FUNCTION "CENTRATORE" : VOID
TITLE =COMANDO CENTRATORE
AUTHOR : D_T
FAMILY : DESTACK
NAME : CENTRAG
VERSION : 0.1

BEGIN
NETWORK
TITLE =Staz.di Centraggio: Comando sblocco
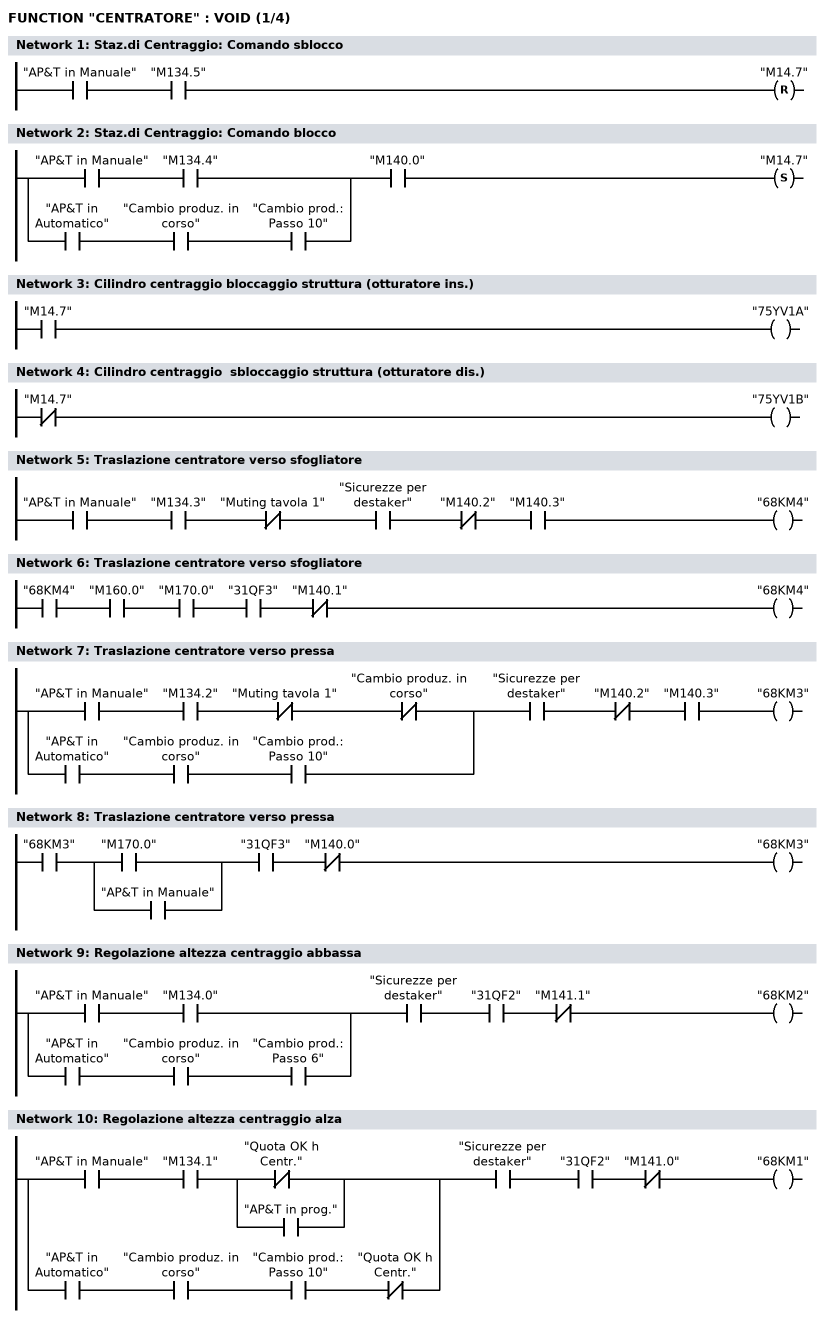
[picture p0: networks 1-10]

      U     "AP&T in Manuale";
      U     "M134.5";
      R     "M14.7";
NETWORK
TITLE =Staz.di Centraggio: Comando blocco

      U(    ;
      U     "AP&T in Manuale";
      U     "M134.4";
      O     ;
      U     "AP&T in Automatico";
      U     "Cambio produz. in corso";
      U     "Cambio prod.: Passo 10";
      )     ;
      U     "M140.0";
      S     "M14.7";
NETWORK
TITLE =Cilindro centraggio bloccaggio struttura (otturatore ins.)

      U     "M14.7";
//      U     "39SQ3"
      =     "75YV1A";
NETWORK
TITLE =Cilindro centraggio  sbloccaggio struttura (otturatore dis.)

      UN    "M14.7";
//      U     "39SQ1"
      =     "75YV1B";
NETWORK
TITLE =Traslazione centratore verso sfogliatore

      U     "AP&T in Manuale";
      U     "M134.3";
      UN    "Muting tavola 1";
      U     "Sicurezze per destaker";
      UN    "M140.2";
      U     "M140.3";
      =     "68KM4";
NETWORK
TITLE =Traslazione centratore verso sfogliatore

      U     "68KM4";
      U     "M160.0";
      U     "M170.0";
      U     "31QF3";
      UN    "M140.1";
      =     "68KM4";
NETWORK
TITLE =Traslazione centratore verso pressa

      U(    ;
      U     "AP&T in Manuale";
      U     "M134.2";
      UN    "Muting tavola 1";
      UN    "Cambio produz. in corso";
      O     ;
      U     "AP&T in Automatico";
      U     "Cambio produz. in corso";
      U     "Cambio prod.: Passo 10";
      )     ;
      U     "Sicurezze per destaker";
      UN    "M140.2";
      U     "M140.3";
      =     "68KM3";
NETWORK
TITLE =Traslazione centratore verso pressa

      U     "68KM3";
      U(    ;
      O     "M170.0";
      O     "AP&T in Manuale";
      )     ;
      U     "31QF3";
      UN    "M140.0";
      =     "68KM3";
NETWORK
TITLE =Regolazione altezza centraggio abbassa

      U(    ;
      U     "AP&T in Manuale";
      U     "M134.0";
      O     ;
      U     "AP&T in Automatico";
      U     "Cambio produz. in corso";
      U     "Cambio prod.: Passo 6";
      )     ;
      U     "Sicurezze per destaker";
      U     "31QF2";
      UN    "M141.1";
      =     "68KM2";
NETWORK
TITLE =Regolazione altezza centraggio alza

      U(    ;
      U     "AP&T in Manuale";
      U     "M134.1";
      U(    ;
      ON    "Quota OK h Centr.";
      O     "AP&T in prog.";
      )     ;
      O     ;
      U     "AP&T in Automatico";
      U     "Cambio produz. in corso";
      U     "Cambio prod.: Passo 10";
      UN    "Quota OK h Centr.";
      )     ;
      U     "Sicurezze per destaker";
      U     "31QF2";
      UN    "M141.0";
      =     "68KM1";
NETWORK
TITLE =

NETWORK
TITLE =Ritardo presenza foglio su centratore
//PER ASSESTAMENTO LAMIERA E RITARDO DEL COMANDO DI CHIUSURA CENTRAGGI
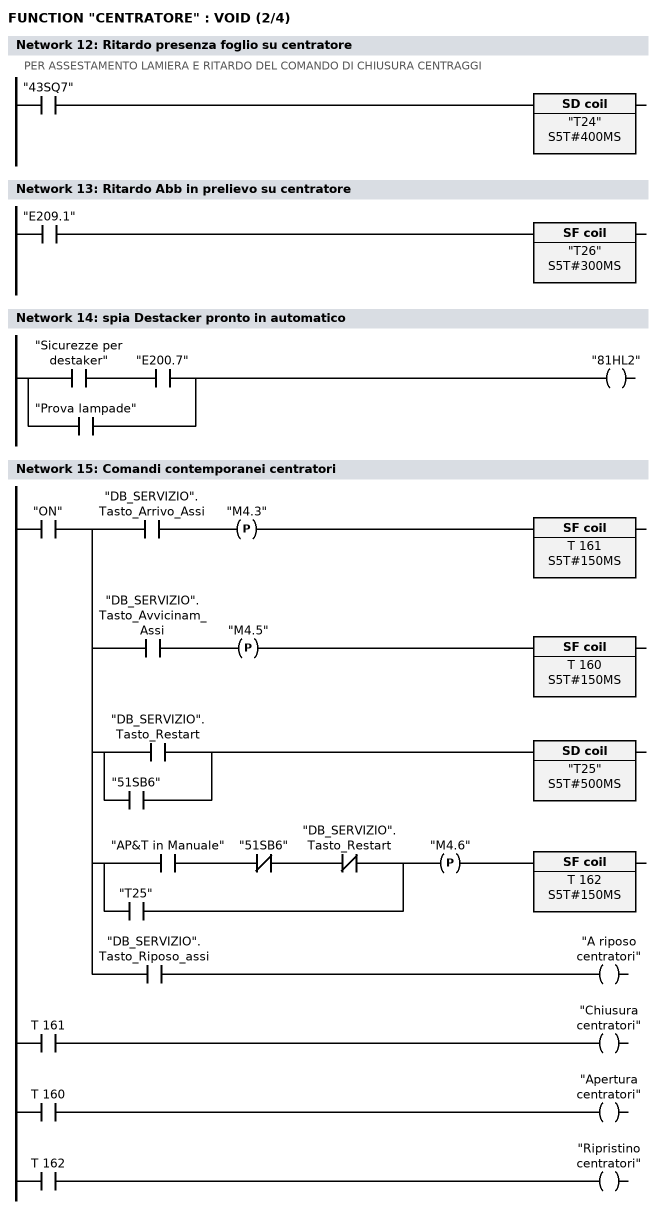
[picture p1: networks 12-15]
      U     "43SQ7";
      L     S5T#400MS;
      SE    "T24";
      NOP   0;
      NOP   0;
      NOP   0;
      NOP   0;
NETWORK
TITLE =Ritardo Abb in prelievo su centratore

      U     "E209.1";
      L     S5T#300MS;
      SA    "T26";
      NOP   0;
      NOP   0;
      NOP   0;
      NOP   0;
NETWORK
TITLE =spia Destacker pronto in automatico

      U     "Sicurezze per destaker";
      U     "E200.7";
      O     "Prova lampade";
      =     "81HL2";
NETWORK
TITLE =Comandi contemporanei centratori

      U     "ON";
      =     L      0.0;
      U     L      0.0;
      U     "DB_SERVIZIO".Tasto_Arrivo_Assi;
      FP    "M4.3";
      L     S5T#150MS;
      SA    T    161;
      NOP   0;
      NOP   0;
      NOP   0;
      U     T    161;
      =     "Chiusura centratori";
      U     L      0.0;
      U     "DB_SERVIZIO".Tasto_Avvicinam_Assi;
      FP    "M4.5";
      L     S5T#150MS;
      SA    T    160;
      NOP   0;
      NOP   0;
      NOP   0;
      U     T    160;
      =     "Apertura centratori";
      U     L      0.0;
      U(    ;
      O     "DB_SERVIZIO".Tasto_Restart;
      O     "51SB6";
      )     ;
      L     S5T#500MS;
      SE    "T25";
      U     L      0.0;
      U(    ;
      U     "AP&T in Manuale";
      UN    "51SB6";
      UN    "DB_SERVIZIO".Tasto_Restart;
      O     "T25";
      )     ;
      FP    "M4.6";
      L     S5T#150MS;
      SA    T    162;
      NOP   0;
      NOP   0;
      NOP   0;
      U     T    162;
      =     "Ripristino centratori";
      U     L      0.0;
      U     "DB_SERVIZIO".Tasto_Riposo_assi;
      =     "A riposo centratori";
NETWORK
TITLE =Comando chiude centraggi
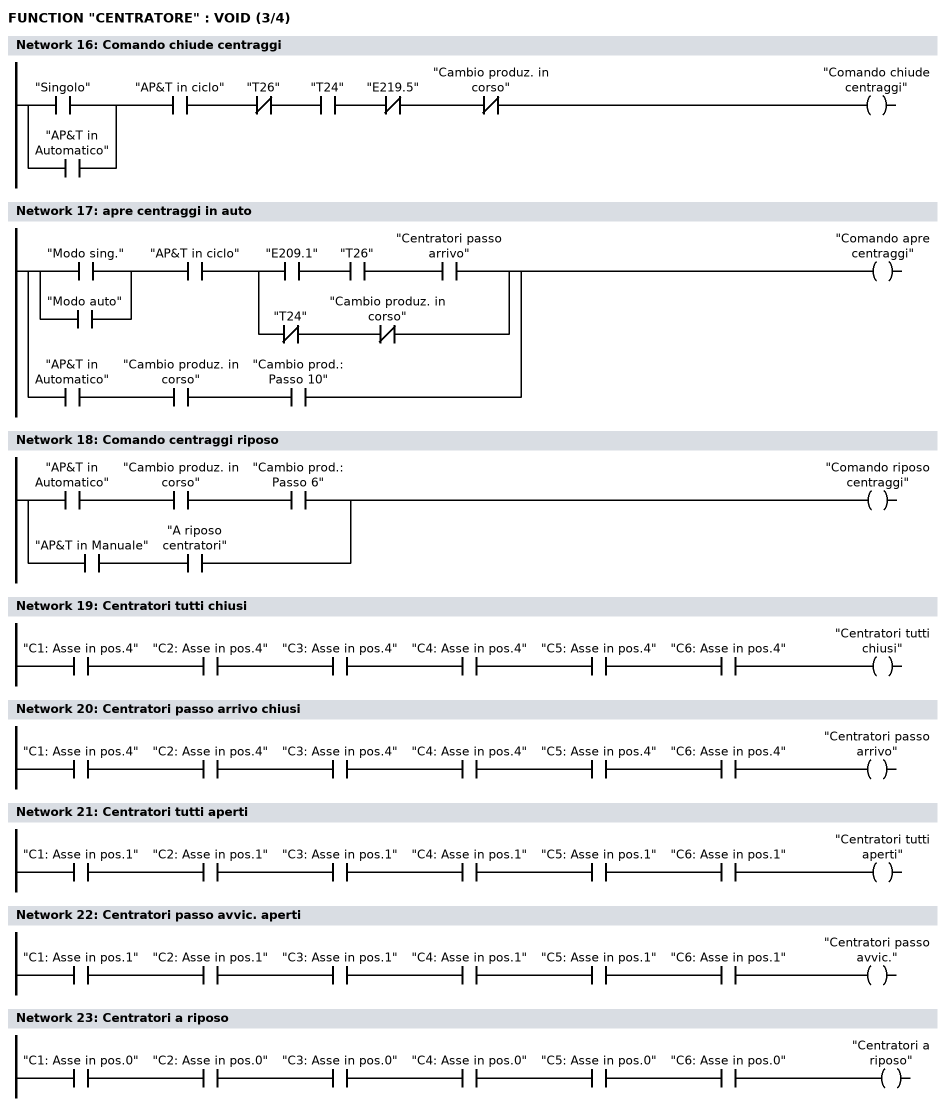
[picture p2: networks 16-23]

      U(    ;
      O     "Singolo";
      O     "AP&T in Automatico";
      )     ;
      U     "AP&T  in ciclo";
      UN    "T26";
      U     "T24";
      UN    "E219.5";
      UN    "Cambio produz. in corso";
      =     "Comando chiude centraggi";
NETWORK
TITLE =apre centraggi in auto

      U(    ;
      O     "Modo sing.";
      O     "Modo auto";
      )     ;
      U     "AP&T  in ciclo";
      U(    ;
      U     "E209.1";
      U     "T26";
      U     "Centratori passo arrivo";
      O     ;
      UN    "T24";
      UN    "Cambio produz. in corso";
      )     ;
      O     ;
      U     "AP&T in Automatico";
      U     "Cambio produz. in corso";
      U     "Cambio prod.: Passo 10";
      =     "Comando apre centraggi";
NETWORK
TITLE =Comando centraggi riposo

      U     "AP&T in Automatico";
      U     "Cambio produz. in corso";
      U     "Cambio prod.: Passo 6";
      O     ;
      U     "AP&T in Manuale";
      U     "A riposo centratori";
      =     "Comando riposo centraggi";
NETWORK
TITLE =Centratori tutti chiusi

      U     "C1: Asse in pos.4";
      U     "C2: Asse in pos.4";
      U     "C3: Asse in pos.4";
      U     "C4: Asse in pos.4";
      U     "C5: Asse in pos.4";
      U     "C6: Asse in pos.4";
      =     "Centratori tutti chiusi";
NETWORK
TITLE =Centratori passo arrivo chiusi

      U     "C1: Asse in pos.4";
      U     "C2: Asse in pos.4";
      U     "C3: Asse in pos.4";
      U     "C4: Asse in pos.4";
      U     "C5: Asse in pos.4";
      U     "C6: Asse in pos.4";
      =     "Centratori passo arrivo";
NETWORK
TITLE =Centratori tutti aperti

      U     "C1: Asse in pos.1";
      U     "C2: Asse in pos.1";
      U     "C3: Asse in pos.1";
      U     "C4: Asse in pos.1";
      U     "C5: Asse in pos.1";
      U     "C6: Asse in pos.1";
      =     "Centratori tutti aperti";
NETWORK
TITLE =Centratori passo avvic. aperti

      U     "C1: Asse in pos.1";
      U     "C2: Asse in pos.1";
      U     "C3: Asse in pos.1";
      U     "C4: Asse in pos.1";
      U     "C5: Asse in pos.1";
      U     "C6: Asse in pos.1";
      =     "Centratori passo avvic.";
NETWORK
TITLE =Centratori a riposo

      U     "C1: Asse in pos.0";
      U     "C2: Asse in pos.0";
      U     "C3: Asse in pos.0";
      U     "C4: Asse in pos.0";
      U     "C5: Asse in pos.0";
      U     "C6: Asse in pos.0";
      =     "Centratori a riposo";
NETWORK
TITLE =
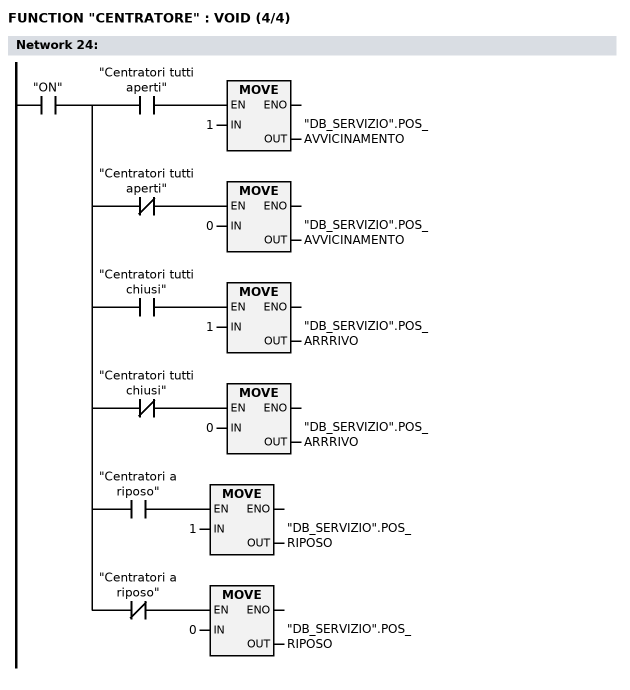
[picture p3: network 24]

      U     "ON";
      =     L      0.0;
      U     L      0.0;
      U     "Centratori tutti aperti";
      SPBNB _001;
      L     1;
      T     "DB_SERVIZIO".POS_AVVICINAMENTO;
_001: NOP   0;
      U     L      0.0;
      UN    "Centratori tutti aperti";
      SPBNB _002;
      L     0;
      T     "DB_SERVIZIO".POS_AVVICINAMENTO;
_002: NOP   0;
      U     L      0.0;
      U     "Centratori tutti chiusi";
      SPBNB _003;
      L     1;
      T     "DB_SERVIZIO".POS_ARRRIVO;
_003: NOP   0;
      U     L      0.0;
      UN    "Centratori tutti chiusi";
      SPBNB _004;
      L     0;
      T     "DB_SERVIZIO".POS_ARRRIVO;
_004: NOP   0;
      U     L      0.0;
      U     "Centratori a riposo";
      SPBNB _005;
      L     1;
      T     "DB_SERVIZIO".POS_RIPOSO;
_005: NOP   0;
      U     L      0.0;
      UN    "Centratori a riposo";
      SPBNB _006;
      L     0;
      T     "DB_SERVIZIO".POS_RIPOSO;
_006: NOP   0;
NETWORK
TITLE =

END_FUNCTION

